(* Logix 5000 AddOnInstructionDefinition export Banner_K50Select_Param_v4; software revision 33.03; part 2 of 2 *)
(* tags used below, declared in another part *)
   K50 : Banner_K50Select_v4;
   Port_Data : Banner_IOL_Port_v4;
   Port : DINT;
   Type : DINT;   // 1=Sensor, 2=Touch, 3=Indicator
   Local_Control : DINT;
   Command_Being_Processed : BOOL;
   Index_Write_Inprocess : INT;
   Inprocess_Index : DINT;
   SP_Index : DINT;   // State Parameters Index
   SP_W_Index : DINT;
(* Banner_K50Select_Param_v4, continued *)

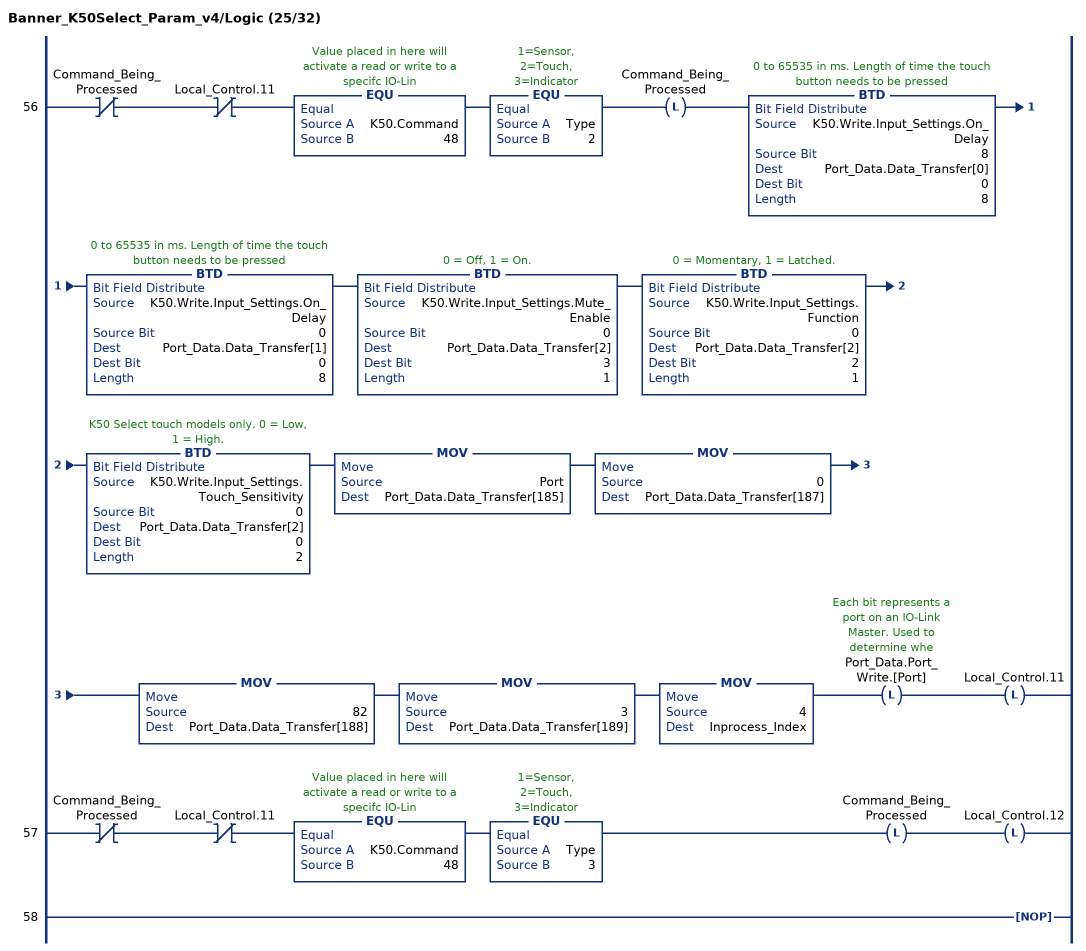
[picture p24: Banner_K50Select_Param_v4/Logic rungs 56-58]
   56: XIO(Command_Being_Processed)XIO(Local_Control.11)EQU(K50.Command,48)EQU(Type,2)OTL(Command_Being_Processed)BTD(K50.Write.Input_Settings.On_Delay,8,Port_Data.Data_Transfer[0],0,8)BTD(K50.Write.Input_Settings.On_Delay,0,Port_Data.Data_Transfer[1],0,8)BTD(K50.Write.Input_Settings.Mute_Enable,0,Port_Data.Data_Transfer[2],3,1)BTD(K50.Write.Input_Settings.Function,0,Port_Data.Data_Transfer[2],2,1)BTD(K50.Write.Input_Settings.Touch_Sensitivity,0,Port_Data.Data_Transfer[2],0,2)MOV(Port,Port_Data.Data_Transfer[185])MOV(0,Port_Data.Data_Transfer[187])MOV(82,Port_Data.Data_Transfer[188])MOV(3,Port_Data.Data_Transfer[189])MOV(4,Inprocess_Index)OTL(Port_Data.Port_Write.[Port])OTL(Local_Control.11);
   57: XIO(Command_Being_Processed)XIO(Local_Control.11)EQU(K50.Command,48)EQU(Type,3)OTL(Command_Being_Processed)OTL(Local_Control.12);
   58: NOP();
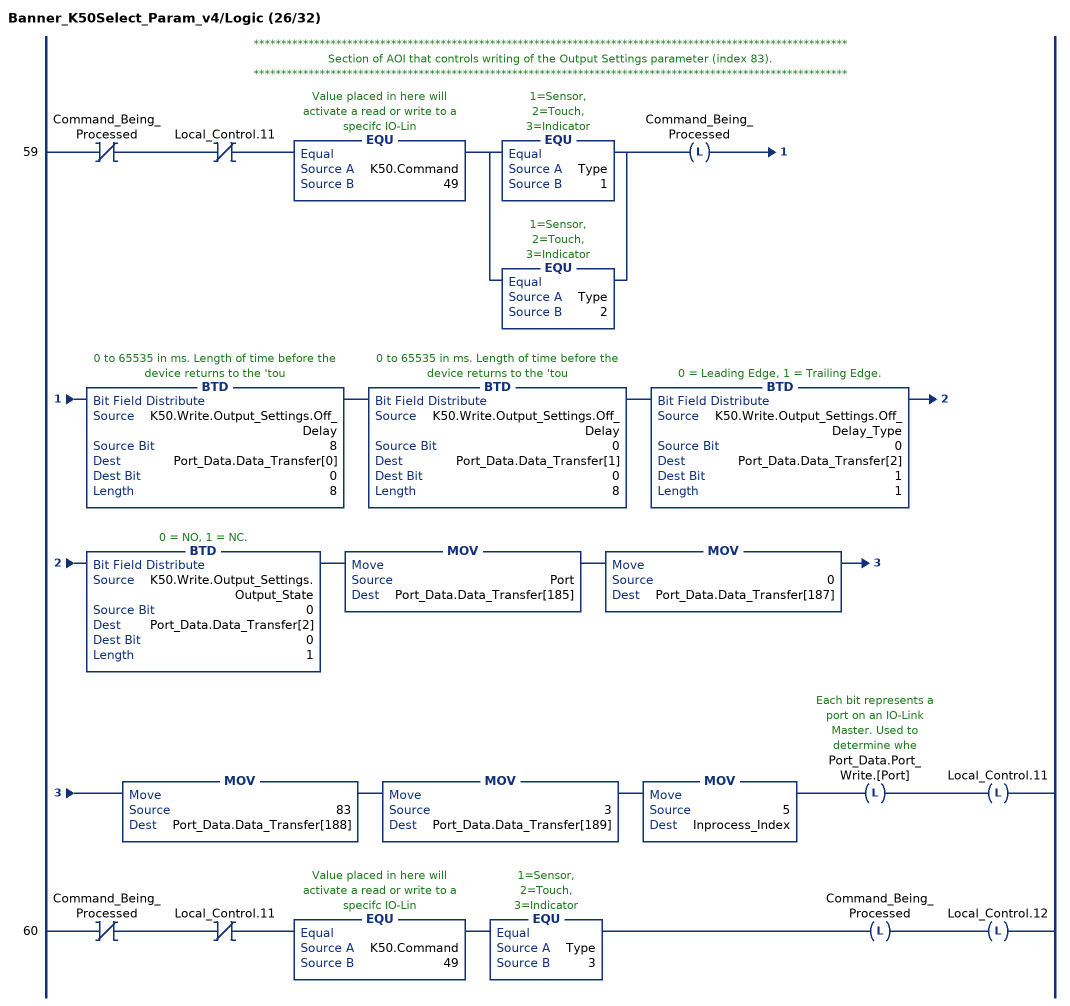
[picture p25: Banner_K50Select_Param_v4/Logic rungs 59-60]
   // ************************************************************************************************************
   // Section of AOI that controls writing of the Output Settings parameter (index 83).
   // ************************************************************************************************************
   59: XIO(Command_Being_Processed)XIO(Local_Control.11)EQU(K50.Command,49)[EQU(Type,1) ,EQU(Type,2) ]OTL(Command_Being_Processed)BTD(K50.Write.Output_Settings.Off_Delay,8,Port_Data.Data_Transfer[0],0,8)BTD(K50.Write.Output_Settings.Off_Delay,0,Port_Data.Data_Transfer[1],0,8)BTD(K50.Write.Output_Settings.Off_Delay_Type,0,Port_Data.Data_Transfer[2],1,1)BTD(K50.Write.Output_Settings.Output_State,0,Port_Data.Data_Transfer[2],0,1)MOV(Port,Port_Data.Data_Transfer[185])MOV(0,Port_Data.Data_Transfer[187])MOV(83,Port_Data.Data_Transfer[188])MOV(3,Port_Data.Data_Transfer[189])MOV(5,Inprocess_Index)OTL(Port_Data.Port_Write.[Port])OTL(Local_Control.11);
   60: XIO(Command_Being_Processed)XIO(Local_Control.11)EQU(K50.Command,49)EQU(Type,3)OTL(Command_Being_Processed)OTL(Local_Control.12);
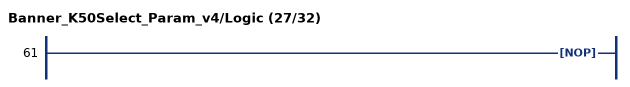
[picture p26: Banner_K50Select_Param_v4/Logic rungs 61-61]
   61: NOP();
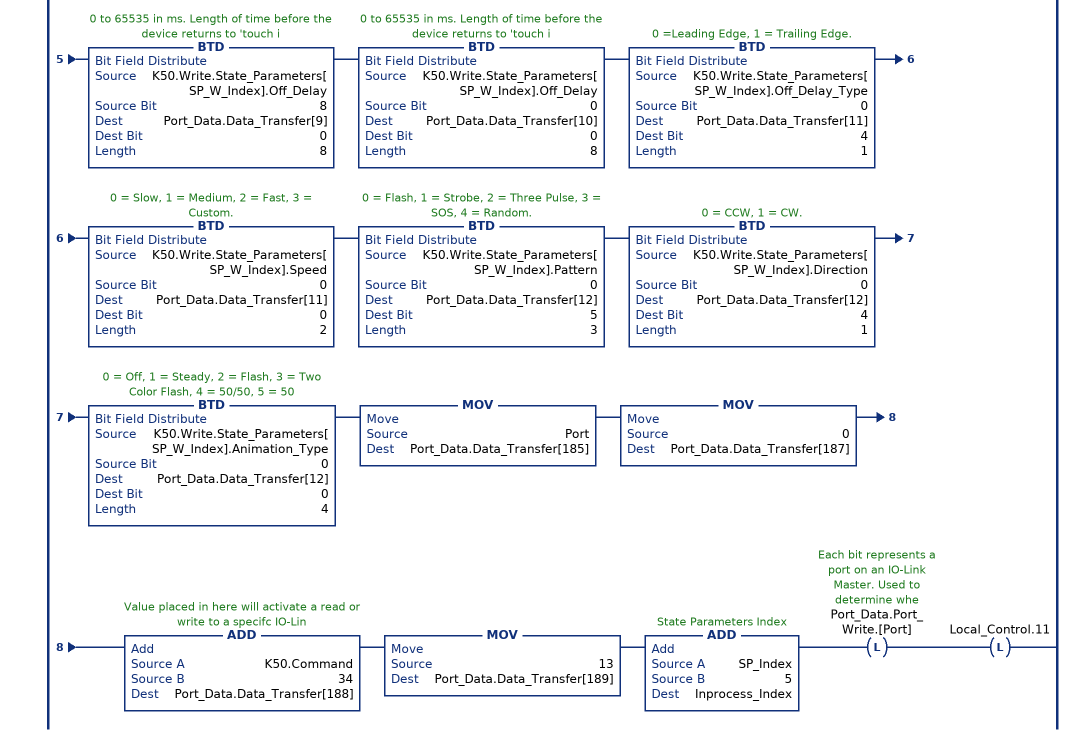
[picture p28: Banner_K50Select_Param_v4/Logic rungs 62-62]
   // ************************************************************************************************************
   // Section of AOI that controls writing of the State Parameters 1 through 5 (indexes 84 through 88).
   // ************************************************************************************************************
   62: XIO(Command_Being_Processed)XIO(Local_Control.11)GEQ(K50.Command,50)LEQ(K50.Command,54)EQU(Type,1)OTL(Command_Being_Processed)SUB(K50.Command,49,SP_W_Index)BTD(K50.Write.State_Parameters[SP_W_Index].Output_State,0,Port_Data.Data_Transfer[0],0,1)BTD(K50.Write.State_Parameters[SP_W_Index].Max_Distance,8,Port_Data.Data_Transfer[1],0,8)BTD(K50.Write.State_Parameters[SP_W_Index].Max_Distance,0,Port_Data.Data_Transfer[2],0,8)BTD(K50.Write.State_Parameters[SP_W_Index].Min_Distance,8,Port_Data.Data_Transfer[3],0,8)BTD(K50.Write.State_Parameters[SP_W_Index].Min_Distance,0,Port_Data.Data_Transfer[4],0,8)BTD(K50.Write.State_Parameters[SP_W_Index].Color_2_Intensity,0,Port_Data.Data_Transfer[5],5,3)BTD(K50.Write.State_Parameters[SP_W_Index].Color_2,0,Port_Data.Data_Transfer[5],0,5)BTD(K50.Write.State_Parameters[SP_W_Index].Color_1_Intensity,0,Port_Data.Data_Transfer[6],5,3)BTD(K50.Write.State_Parameters[SP_W_Index].Color_1,0,Port_Data.Data_Transfer[6],0,5)BTD(K50.Write.State_Parameters[SP_W_Index].Sequence_Start_Location,0,Port_Data.Data_Transfer[7],0,8)BTD(K50.Write.State_Parameters[SP_W_Index].Static_Sequence,0,Port_Data.Data_Transfer[8],0,8)BTD(K50.Write.State_Parameters[SP_W_Index].Off_Delay,8,Port_Data.Data_Transfer[9],0,8)BTD(K50.Write.State_Parameters[SP_W_Index].Off_Delay,0,Port_Data.Data_Transfer[10],0,8)BTD(K50.Write.State_Parameters[SP_W_Index].Off_Delay_Type,0,Port_Data.Data_Transfer[11],4,1)BTD(K50.Write.State_Parameters[SP_W_Index].Speed,0,Port_Data.Data_Transfer[11],0,2)BTD(K50.Write.State_Parameters[SP_W_Index].Pattern,0,Port_Data.Data_Transfer[12],5,3)BTD(K50.Write.State_Parameters[SP_W_Index].Direction,0,Port_Data.Data_Transfer[12],4,1)BTD(K50.Write.State_Parameters[SP_W_Index].Animation_Type,0,Port_Data.Data_Transfer[12],0,4)MOV(Port,Port_Data.Data_Transfer[185])MOV(0,Port_Data.Data_Transfer[187])ADD(K50.Command,34,Port_Data.Data_Transfer[188])MOV(13,Port_Data.Data_Transfer[189])ADD(SP_Index,5,Inprocess_Index)OTL(Port_Data.Port_Write.[Port])OTL(Local_Control.11);
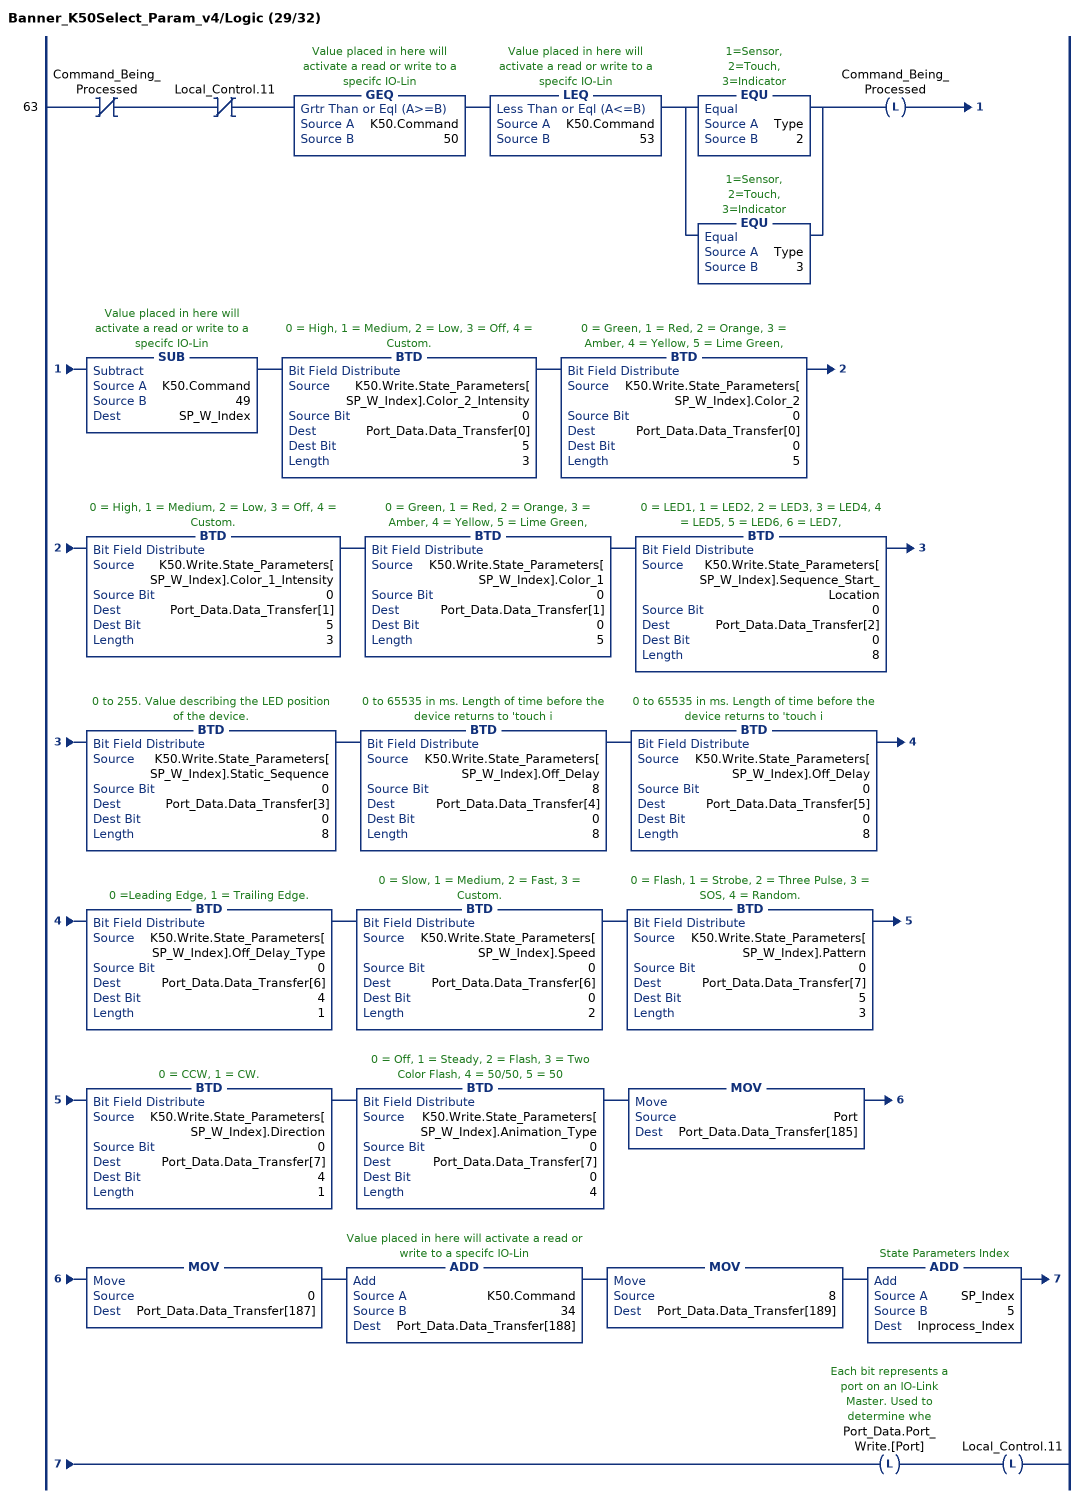
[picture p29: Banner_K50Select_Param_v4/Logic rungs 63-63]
   63: XIO(Command_Being_Processed)XIO(Local_Control.11)GEQ(K50.Command,50)LEQ(K50.Command,53)[EQU(Type,2) ,EQU(Type,3) ]OTL(Command_Being_Processed)SUB(K50.Command,49,SP_W_Index)BTD(K50.Write.State_Parameters[SP_W_Index].Color_2_Intensity,0,Port_Data.Data_Transfer[0],5,3)BTD(K50.Write.State_Parameters[SP_W_Index].Color_2,0,Port_Data.Data_Transfer[0],0,5)BTD(K50.Write.State_Parameters[SP_W_Index].Color_1_Intensity,0,Port_Data.Data_Transfer[1],5,3)BTD(K50.Write.State_Parameters[SP_W_Index].Color_1,0,Port_Data.Data_Transfer[1],0,5)BTD(K50.Write.State_Parameters[SP_W_Index].Sequence_Start_Location,0,Port_Data.Data_Transfer[2],0,8)BTD(K50.Write.State_Parameters[SP_W_Index].Static_Sequence,0,Port_Data.Data_Transfer[3],0,8)BTD(K50.Write.State_Parameters[SP_W_Index].Off_Delay,8,Port_Data.Data_Transfer[4],0,8)BTD(K50.Write.State_Parameters[SP_W_Index].Off_Delay,0,Port_Data.Data_Transfer[5],0,8)BTD(K50.Write.State_Parameters[SP_W_Index].Off_Delay_Type,0,Port_Data.Data_Transfer[6],4,1)BTD(K50.Write.State_Parameters[SP_W_Index].Speed,0,Port_Data.Data_Transfer[6],0,2)BTD(K50.Write.State_Parameters[SP_W_Index].Pattern,0,Port_Data.Data_Transfer[7],5,3)BTD(K50.Write.State_Parameters[SP_W_Index].Direction,0,Port_Data.Data_Transfer[7],4,1)BTD(K50.Write.State_Parameters[SP_W_Index].Animation_Type,0,Port_Data.Data_Transfer[7],0,4)MOV(Port,Port_Data.Data_Transfer[185])MOV(0,Port_Data.Data_Transfer[187])ADD(K50.Command,34,Port_Data.Data_Transfer[188])MOV(8,Port_Data.Data_Transfer[189])ADD(SP_Index,5,Inprocess_Index)OTL(Port_Data.Port_Write.[Port])OTL(Local_Control.11);
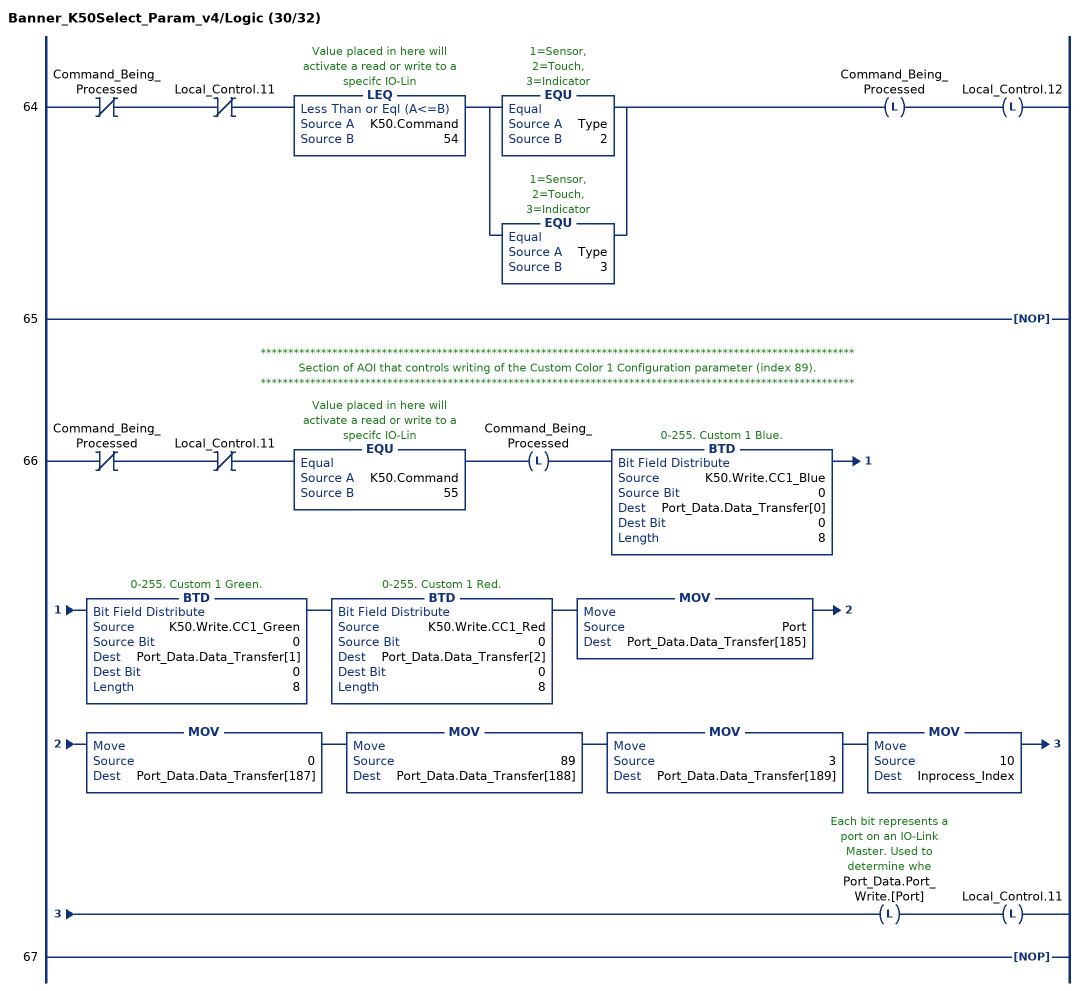
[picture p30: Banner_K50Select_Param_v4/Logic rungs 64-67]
   64: XIO(Command_Being_Processed)XIO(Local_Control.11)LEQ(K50.Command,54)[EQU(Type,2) ,EQU(Type,3) ]OTL(Command_Being_Processed)OTL(Local_Control.12);
   65: NOP();
   // ************************************************************************************************************
   // Section of AOI that controls writing of the Custom Color 1 Configuration parameter (index 89).
   // ************************************************************************************************************
   66: XIO(Command_Being_Processed)XIO(Local_Control.11)EQU(K50.Command,55)OTL(Command_Being_Processed)BTD(K50.Write.CC1_Blue,0,Port_Data.Data_Transfer[0],0,8)BTD(K50.Write.CC1_Green,0,Port_Data.Data_Transfer[1],0,8)BTD(K50.Write.CC1_Red,0,Port_Data.Data_Transfer[2],0,8)MOV(Port,Port_Data.Data_Transfer[185])MOV(0,Port_Data.Data_Transfer[187])MOV(89,Port_Data.Data_Transfer[188])MOV(3,Port_Data.Data_Transfer[189])MOV(10,Inprocess_Index)OTL(Port_Data.Port_Write.[Port])OTL(Local_Control.11);
   67: NOP();
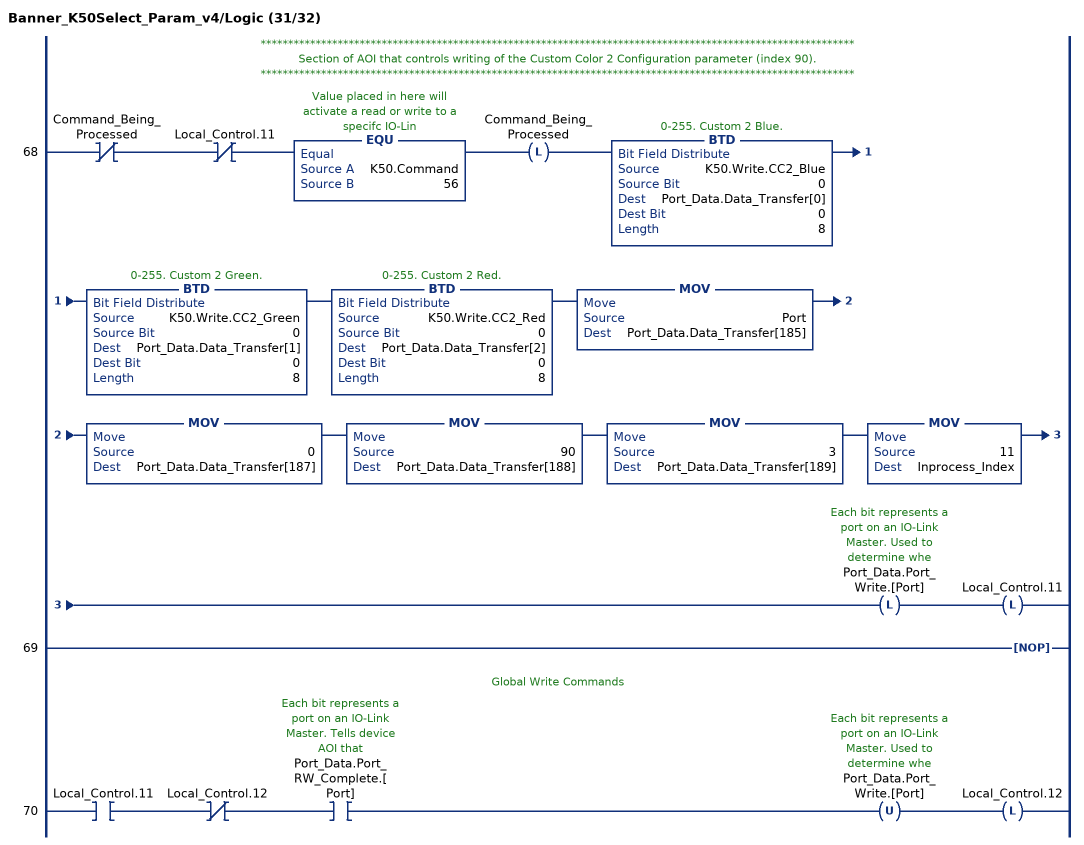
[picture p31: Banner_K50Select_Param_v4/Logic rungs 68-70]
   // ************************************************************************************************************
   // Section of AOI that controls writing of the Custom Color 2 Configuration parameter (index 90).
   // ************************************************************************************************************
   68: XIO(Command_Being_Processed)XIO(Local_Control.11)EQU(K50.Command,56)OTL(Command_Being_Processed)BTD(K50.Write.CC2_Blue,0,Port_Data.Data_Transfer[0],0,8)BTD(K50.Write.CC2_Green,0,Port_Data.Data_Transfer[1],0,8)BTD(K50.Write.CC2_Red,0,Port_Data.Data_Transfer[2],0,8)MOV(Port,Port_Data.Data_Transfer[185])MOV(0,Port_Data.Data_Transfer[187])MOV(90,Port_Data.Data_Transfer[188])MOV(3,Port_Data.Data_Transfer[189])MOV(11,Inprocess_Index)OTL(Port_Data.Port_Write.[Port])OTL(Local_Control.11);
   69: NOP();
   // Global Write Commands
   70: XIC(Local_Control.11)XIO(Local_Control.12)XIC(Port_Data.Port_RW_Complete.[Port])OTU(Port_Data.Port_Write.[Port])OTL(Local_Control.12);
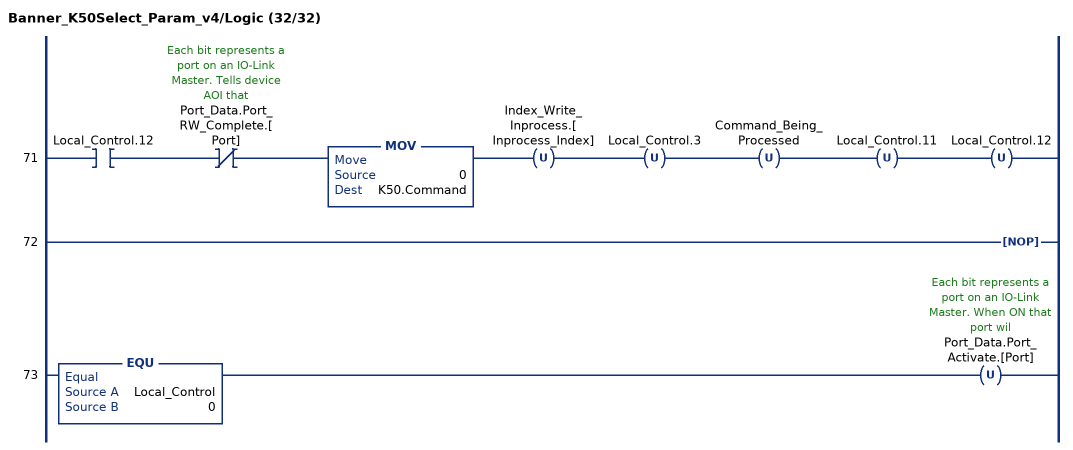
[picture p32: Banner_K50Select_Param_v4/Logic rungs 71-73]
   71: XIC(Local_Control.12)XIO(Port_Data.Port_RW_Complete.[Port])MOV(0,K50.Command)OTU(Index_Write_Inprocess.[Inprocess_Index])OTU(Local_Control.3)OTU(Command_Being_Processed)OTU(Local_Control.11)OTU(Local_Control.12);
   72: NOP();
   73: EQU(Local_Control,0)OTU(Port_Data.Port_Activate.[Port]);
END_ROUTINE
END_ADD_ON_INSTRUCTION
